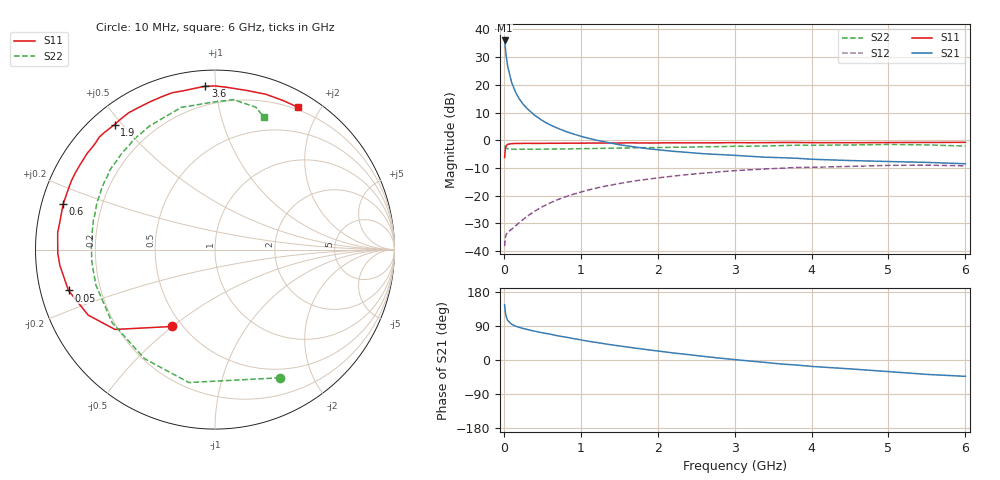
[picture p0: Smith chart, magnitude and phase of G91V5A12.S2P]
! SIEMENS Small Signal Semiconductors
! BFG235
! Si NPN RF Bipolar Junction Transistor in SOT223
! VCE = 1.5 V  IC = 120 mA
! Common Emitter S-Parameters:  July  1994
# GHz  S  MA  R  50
!  f  S11  S21  S12  S22
! GHz  MAG  ANG  MAG  ANG  MAG  ANG  MAG  ANG
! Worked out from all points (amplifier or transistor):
!   40 points, 10 MHz to 6 GHz, reference 50 ohm
!   highest |S21| = 36.0 dB at 10 MHz (marker M1)
!   |S21| within 3 dB of that: start of sweep to 20.57 MHz
!   unconditionally stable (mu >= 1): 429.6 MHz to 1.586 GHz; 1.742 GHz to 1.95 GHz
!   at 200 MHz: K = 0.81, MSG = 22.3 dB, |S12| = -29.7 dB
!   at 1.5 GHz: K = 1.02, MAG = 6.2 dB, |S12| = -15.6 dB
!   at 6 GHz: K = 0.94, MSG = 0.4 dB, |S12| = -9.2 dB
!   S11 on the Smith chart (normalised r, x): 10 MHz: 0.44, -0.50; 50 MHz: 0.08, -0.14; 600 MHz: 0.06, +0.15; 1.9 GHz: 0.07, +0.48; 3.6 GHz: 0.09, +0.94; 6 GHz: 0.17, +1.73
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0.01  0.4896 -119.0  63.14 145.6  0.0123 56.2  0.8008 -63.1
0.02  0.7131 -141.4  45.47 125.6  0.0176 40.0  0.7548 -101.1
0.03  0.7955 -152.7  33.77 114.8  0.0198 34.2  0.7235 -122.9
0.05  0.8473 -164.4  21.61 104.3  0.022 29.4  0.7028 -144.6
0.1  0.8688 -174.1  11.17 94.6  0.0247 34.5  0.6925 -163.4
0.15  0.8763 -178.7  7.473 89.5  0.0283 41.5  0.6882 -171.0
0.2  0.8764 178.7  5.591 86.2  0.0327 46.9  0.6898 -175.3
0.25  0.8787 175.9  4.502 83.2  0.0372 50.7  0.6874 -178.3
0.3  0.8816 173.8  3.76 80.8  0.0421 53.6  0.6891 179.0
0.4  0.8779 169.6  2.834 76.0  0.0525 56.7  0.6876 175.3
0.5  0.8796 166.3  2.268 71.8  0.0632 58.3  0.6909 172.1
0.6  0.8833 163.3  1.9 68.3  0.074 58.7  0.6936 169.1
0.8  0.8844 157.1  1.45 60.5  0.0956 57.4  0.6971 163.8
1.1  0.8884 148.1  1.084 49.4  0.1268 53.4  0.7095 156.7
1.5  0.8921 138.3  0.831 37.2  0.1657 46.5  0.724 147.7
1.9  0.893 128.8  0.698 26.2  0.2009 39.1  0.7367 139.5
2.2  0.9016 122.2  0.633 18.6  0.2256 33.3  0.748 133.6
3.2  0.9023 101.2  0.514 -2.8  0.2932 13.9  0.7822 114.8
3.6  0.912 93.4  0.485 -10.5  0.3135 5.7  0.8006 106.8
4.5  0.9043 78.4  0.431 -23.4  0.3377 -9.8  0.821 91.3
5.5  0.913 65.6  0.399 -38.0  0.3556 -27.3  0.8251 74.0
6  0.9177 59.8  0.377 -43.1  0.3457 -33.8  0.7865 69.6
